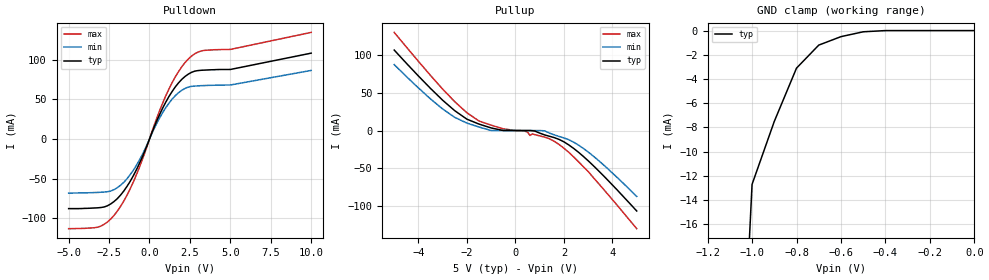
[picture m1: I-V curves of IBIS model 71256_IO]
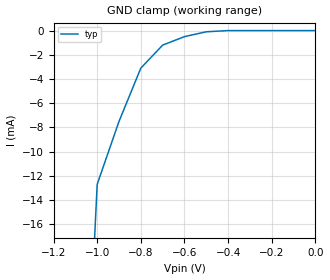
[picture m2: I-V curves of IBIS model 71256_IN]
[IBIS Ver]   1.1
[File name]   idt71256.ibs
[File Rev]   1.1
[Date]   11/25/96
[Source]   Integrated Device Technology
[Notes]   Some versions of this part may have power clamping
|   on the I/Os, which is not included in this model.
[Disclaimer]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
[Component]   IDT71256
|   Includes S, L, SA and LA versions
[Manufacturer]   Integrated Device Technology
[Package]
|   PJ28 (300-mil SOJ)
|   typ   min   max
R_pkg   100.0m   NA   NA
L_pkg   8nH   6nH   12nH
C_pkg   1.2pF   0.8pF   1.5pF
[Pin]   signal_name   model_name   R_pin   L_pin   C_pin
1   A14   71256_IN
2   A12   71256_IN
3   A7   71256_IN
4   A6   71256_IN
5   A5   71256_IN
6   A4   71256_IN
7   A3   71256_IN
8   A2   71256_IN
9   A1   71256_IN
10   A0   71256_IN
11   I/O0   71256_IO
12   I/O1   71256_IO
13   I/O2   71256_IO
14   GND   GND
15   I/O3   71256_IO
16   I/O4   71256_IO
17   I/O5   71256_IO
18   I/O6   71256_IO
19   I/O7   71256_IO
20   CS#   71256_IN
21   A10   71256_IN
22   OE#   71256_IN
23   A11   71256_IN
24   A9   71256_IN
25   A8   71256_IN
26   A13   71256_IN
27   WE#   71256_IN
28   Vcc   POWER
| Models and submodels in the file (2): 71256_IO (I/O), 71256_IN (Input)
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|   71256_IO MODEL
[MODEL]   71256_IO
Model_type   I/O
Polarity   Non-Inverting
Enable   Active-Low
|   Signals   I/O [7:0]
Vinl = 0.8V
Vinh = 2.2V
|   typ   min   max
C_comp   3.5pF   NA   NA
|   typ   min   max
[Voltage range]   5.0V   4.5V   5.5V
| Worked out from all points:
|   slope of the pulldown table from 0 to 0.75 V, typ, clamps not added: 20.7 ohm
|   slope of the pullup table from 0 to 0.75 V, typ, clamps not added: 1.5 kohm
|   GND clamp passes 1 mA (typ) near -0.67 V on its own axis
[Pulldown]
|   V_ol (volts)   I_typ   I_min   I_max
-5V       -87.8mA    -68.2mA    -113.1mA
-3V       -86.4mA    -67.1mA    -109.8mA
-2V       -75.4mA    -61.6mA    -91.3mA
-1.4V     -60mA      -50.4mA    -71.2mA
-800mV    -38.4mA    -32.9mA    -44.6mA
600mV     29.8mA     25.7mA     34.5mA
1.2V      53.6mA     45mA       63mA
2V        75.4mA     61.6mA     91.3mA
2.6V      84.2mA     66.5mA     104.7mA
3.4V      87mA       67.5mA     111.9mA
5V        87.8mA     68.2mA     113.1mA
10V       108.4mA    86.6mA     134.6mA
[GND_clamp]
|   Voltage   I_typ   I_min   I_max
-5V       -1.52A     NA         NA
-1V       -12.7mA    NA         NA
-900mV    -7.5mA     NA         NA
-800mV    -3.1mA     NA         NA
-700mV    -1.2mA     NA         NA
-600mV    -500uA     NA         NA
-500mV    -100uA     NA         NA
-400mV    0A         NA         NA
-300mV    0A         NA         NA
-200mV    0A         NA         NA
-100mV    0A         NA         NA
0V        0A         NA         NA
[Pullup]
|   V_oh (volts)   I_typ   I_min   I_max
-5V       106.6mA    87.3mA     130mA
-3V       40.1mA     28.5mA     54.8mA
-2V       15mA       9.8mA      23.5mA
-1.5V     8.5mA      4.6mA      12.6mA
-1V       3.4mA      0A         7.1mA
600mV     0A         0A         -6.5mA
800mV     -700uA     0A         -5.5mA
1.4V      -7.6mA     -3.3mA     -10.9mA
2V        -15mA      -9.8mA     -23.5mA
2.6V      -28.8mA    -19.3mA    -41.3mA
3.2V      -46.2mA    -33.6mA    -61.9mA
5V        -106.6mA   -87.3mA    -130mA
[POWER_clamp]
|   Voltage   I_typ   I_min   I_max
-5V       0A         NA         NA
-4V       0A         NA         NA
-3V       0A         NA         NA
0V        0A         NA         NA
[Ramp]
|   typ   min   max
dV/dt_r   1.2/0.9n   0.9/1.0n   1.5/0.8n
dV/dt_f   2.0/1.4n   1.7/1.5n   2.3/1.2n
[MODEL]   71256_IN
Model_type   Input
Polarity   Non-Inverting
Enable   Active-Low
Vinl = 0.8V
Vinh = 2.2V
|   typ   min   max
C_comp   2.5pF   NA   NA
|   typ   min   max
[Voltage range]   5.0V   4.5V   5.5V
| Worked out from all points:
|   GND clamp passes 1 mA (typ) near -0.67 V on its own axis
[GND_clamp]
|   Voltage   I_typ   I_min   I_max
-5V       -1.52A     NA         NA
-1V       -12.7mA    NA         NA
-900mV    -7.5mA     NA         NA
-800mV    -3.1mA     NA         NA
-700mV    -1.2mA     NA         NA
-600mV    -500uA     NA         NA
-500mV    -100uA     NA         NA
-400mV    0A         NA         NA
-300mV    0A         NA         NA
-200mV    0A         NA         NA
-100mV    0A         NA         NA
0V        0A         NA         NA
[POWER_clamp]
|   Voltage   I_typ   I_min   I_max
-5V       0A         NA         NA
-4V       0A         NA         NA
-3V       0A         NA         NA
0V        0A         NA         NA
